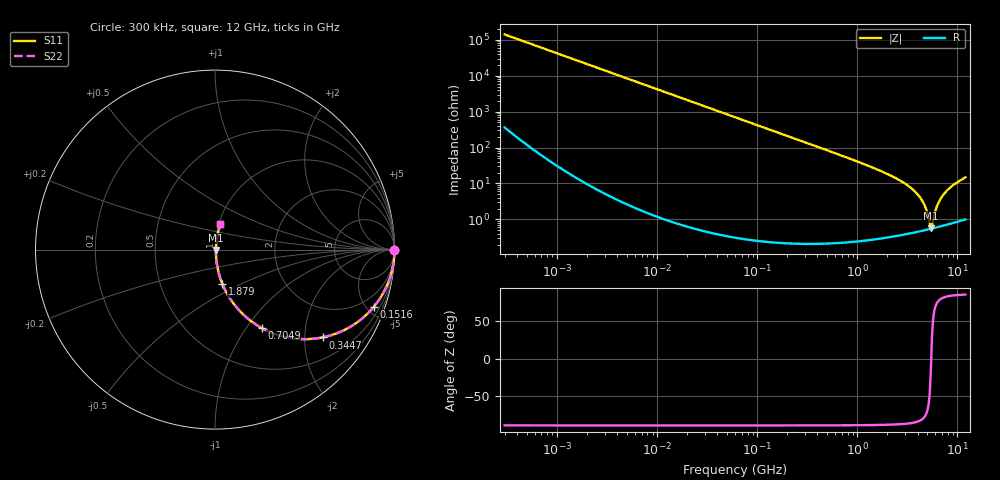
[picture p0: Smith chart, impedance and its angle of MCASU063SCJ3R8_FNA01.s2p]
! MCASU063SCJ3R8_FNA01  S-PARAMETER MODEL  ( General Type )
! Model Generated by TAIYO YUDEN Corporation (http://www.ty-top.com)
! Version 1.0
! TAIYO YUDEN Control No. 130801
! Copyright(c) 2013 TAIYO YUDEN CO.,LTD. All Rights Reserved.
! Product Description (link to TY-COMPAS)
! https://ds.yuden.co.jp/TYCOMPAS/or/detail?pn=MCASU063SCJ3R8CFNA01&u=M
! Products Name : Multilayer Ceramic Capacitors
! Characteristics :
!  Capacitance : 3.8 pF , Rated Voltage : 50V , TCC : CJ / C0J
!  Case Size : 0.6 x 0.3 / 0.024 x 0.012 [mm/inch] , Thickness : 0.3 / 0.012 [mm/inch]
!  (Conditions: Temperature = 25 degC , DC Bias Current/Voltage = 0A / 0V)
! External Node Assignments :
!  1  o---| |---o  2
! GND o---------o GND
! Frequency Range : 0.3MHz  -  12000MHz  [ 401 STEP ]
# MHz S RI R 50
! Freq[MHz].  S11 Real  S11 Imag  S21 Real  S21 Imag  S12 Real  S12 Imag  S22 Real  S22 Imag
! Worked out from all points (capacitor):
!   401 points, 300 kHz to 12 GHz, reference 50 ohm
!   read as one part in series: C = 3.76 pF near 316.3 kHz
!   lowest |Z| = 571 mohm at 5.42 GHz (marker M1)
!   series resonance near 5.469 GHz, so ESL is about 230 pH
!   S11 on the Smith chart (normalised r, x): 300 kHz: open; 151.6 MHz: 1.00, -5.58; 344.7 MHz: 1.00, -2.45; 704.9 MHz: 1.00, -1.18; 1.879 GHz: 1.01, -0.40; 12 GHz: 1.02, +0.30
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0.3  1 -0.000709  2.33e-06 0.000709  2.33e-06 0.000709  1 -0.000709
1.769972  1 -0.00418  1.95e-05 0.00418  1.95e-05 0.00418  1 -0.00418
10.44266  0.9994 -0.0247  0.000615 0.0247  0.000615 0.0247  0.9994 -0.0247
60  0.9802 -0.139  0.0198 0.139  0.0198 0.139  0.9802 -0.139
151.6462  0.8859 -0.3175  0.1141 0.3175  0.1141 0.3175  0.8859 -0.3175
344.7396  0.5991 -0.4892  0.4009 0.4892  0.4009 0.4892  0.5991 -0.4892
353.9943  0.5863 -0.4916  0.4137 0.4916  0.4137 0.4916  0.5863 -0.4916
704.9044  0.2594 -0.4364  0.7406 0.4364  0.7406 0.4364  0.2594 -0.4364
1105.905  0.1205 -0.3222  0.8795 0.3222  0.8795 0.3222  0.1205 -0.3222
1878.541  0.0408 -0.1902  0.9592 0.1902  0.9592 0.1902  0.0408 -0.1902
2088.533  0.0321 -0.1672  0.9679 0.1672  0.9679 0.1672  0.0321 -0.1672
3026.31  0.0131 -0.0957  0.9869 0.0957  0.9869 0.0957  0.0131 -0.0957
3944.255  0.00711 -0.0513  0.9929 0.0513  0.9929 0.0513  0.00711 -0.0513
4623.766  0.00561 -0.0263  0.9944 0.0263  0.9944 0.0263  0.00561 -0.0263
5278.635  0.00539 -0.00598  0.9946 0.00598  0.9946 0.00598  0.00539 -0.00598
5420.343  0.00545 -0.0016  0.9945 0.0016  0.9945 0.0016  0.00545 -0.0016
5715.274  0.00571 0.00756  0.9943 -0.00756  0.9943 -0.00756  0.00571 0.00756
6188.031  0.0064 0.0208  0.9936 -0.0208  0.9936 -0.0208  0.0064 0.0208
6524.734  0.00707 0.0295  0.9929 -0.0295  0.9929 -0.0295  0.00707 0.0295
7254.098  0.009 0.0479  0.991 -0.0479  0.991 -0.0479  0.009 0.0479
8966.534  0.0153 0.0859  0.9847 -0.0859  0.9847 -0.0859  0.0153 0.0859
12000  0.0306 0.1418  0.9694 -0.1418  0.9694 -0.1418  0.0306 0.1418
